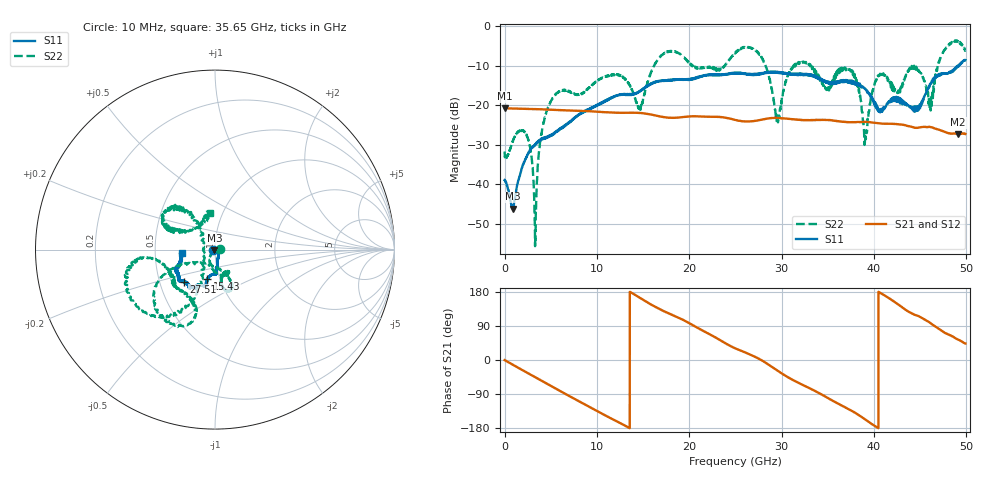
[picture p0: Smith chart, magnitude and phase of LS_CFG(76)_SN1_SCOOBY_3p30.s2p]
!Keysight Technologies,N5245B,MY58422026,A.13.80.08
!Date: Thursday, March 19, 2020 23:50:51
!Correction: S11(Full 2 Port(1,2))
!S21(Full 2 Port(1,2))
!S12(Full 2 Port(1,2))
!S22(Full 2 Port(1,2))
!S2P File: Measurements: S11, S21, S12, S22:
# Hz S DB R 50.0
!freq dBS11 angS11 dBS21 angS21 dBS12 angS12 dBS22 angS22
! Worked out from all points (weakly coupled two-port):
!   4991 points, 10 MHz to 49.91 GHz, reference 50 ohm
!   highest |S21| = -20.74 dB at 10 MHz (marker M1); lowest = -27.3 dB at 49.11 GHz (marker M2)
!   lowest |S11| = -46.1 dB at 870 MHz (marker M3), VSWR 1.01, Z = 49.7 - j0.385 ohm
!   |S11| at or under -10 dB: start of sweep to 49.12 GHz; 49.16969 GHz to 49.22302 GHz (53.33 MHz wide, 0.108 % of centre)
!   |S22| runs from -55.6 to -3.6 dB; largest |S21 - S12| = 0.00091
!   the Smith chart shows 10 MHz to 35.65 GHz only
!   S11 on the Smith chart (normalised r, x): 10 MHz: 0.98, -0.01; 15.43 GHz: 0.87, -0.30; 27.51 GHz: 0.66, -0.25; 35.65 GHz: 0.69, -0.02
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1e7  -38.91 -165.8  -20.74 -0.2  -20.74 -0.3  -31.70 1.7
8.7e8  -46.14 -128.2  -20.82 -12.1  -20.81 -12.1  -29.25 -27.0
2.44e9  -32.76 -53.9  -20.92 -33.6  -20.90 -33.5  -27.93 15.4
3.33e9  -29.79 -55.5  -20.98 -45.6  -20.97 -45.6  -54.29 124.8
4.82e9  -27.99 -61.5  -21.11 -66.0  -21.10 -65.9  -19.81 -101.4
8.33e9  -22.10 -80.3  -21.41 -112.7  -21.41 -112.6  -17.11 -69.1
1.543e10  -15.34 -104.4  -22.16 152.8  -22.16 152.9  -14.88 -155.5
1.665e10  -13.99 -104.0  -22.73 136.0  -22.72 136.1  -8.30 -148.1
2.496e10  -11.94 -124.4  -23.67 31.1  -23.66 31.3  -6.88 -170.5
2.751e10  -12.01 -134.4  -23.80 3.7  -23.80 3.9  -6.76 -125.1
2.956e10  -11.60 -141.0  -23.21 -28.3  -23.20 -28.0  -23.42 -178.5
3.103e10  -12.05 -145.9  -23.50 -50.2  -23.52 -49.9  -10.77 128.6
3.328e10  -12.44 -155.9  -23.74 -77.7  -23.74 -77.3  -10.44 156.4
3.565e10  -14.64 -174.6  -23.85 -109.0  -23.79 -108.5  -13.68 98.0
3.78e10  -14.49 178.0  -24.29 -136.9  -24.24 -137.0  -11.81 135.0
3.905e10  -15.77 174.0  -24.20 -156.6  -24.19 -156.8  -29.23 -126.5
4.024e10  -20.43 156.9  -24.48 -176.2  -24.47 -176.4  -13.64 -4.0
4.16e10  -19.06 108.5  -24.68 163.7  -24.70 163.7  -13.92 25.8
4.445e10  -20.87 56.4  -25.70 119.0  -25.72 119.3  -10.23 -15.4
4.614e10  -14.53 8.5  -25.49 97.0  -25.50 97.2  -20.90 -45.2
4.911e10  -10.13 -12.8  -27.31 53.8  -27.32 53.8  -3.81 -44.3
4.991e10  -8.58 -13.3  -27.23 43.4  -27.26 43.5  -6.16 -29.1
